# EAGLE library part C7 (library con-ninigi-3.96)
NINIGI
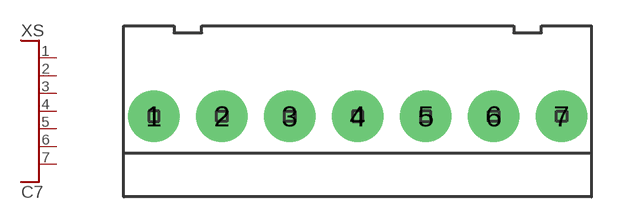
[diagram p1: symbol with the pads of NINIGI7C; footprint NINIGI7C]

Designator prefix XS

## C7  [NINIGI7C]
1  P$1
2  P$2
3  P$3
4  P$4
5  P$5
6  P$6
7  P$7

## Footprint NINIGI7C (pad centres in mm)
drill 1.6 pad 3: 1 -11.88,0; 2 -7.92,0; 3 -3.96,0; 4 0,0; 5 3.96,0; 6 7.92,0; 7 11.88,0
